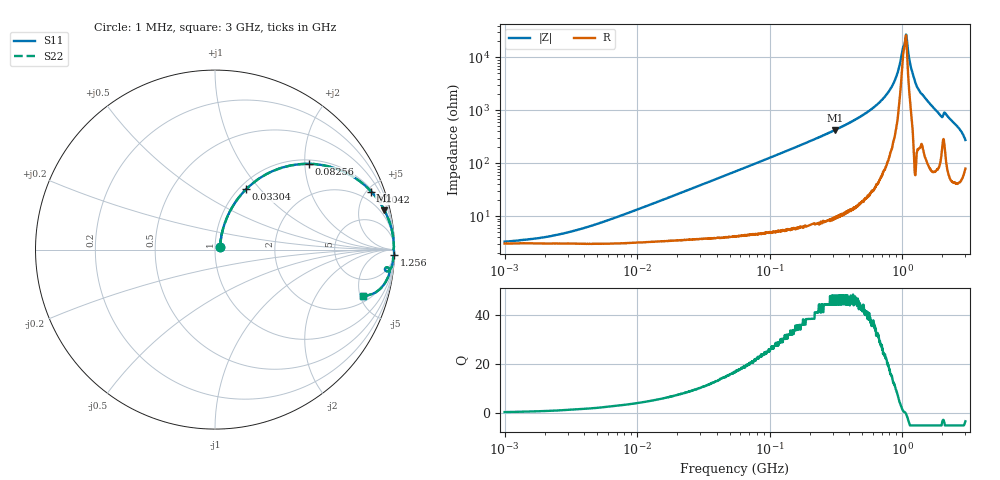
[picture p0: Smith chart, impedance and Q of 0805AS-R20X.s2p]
!s-Parameter Generated by FASTRON Sdn. Bhd.
!FASTRON P/N : 0805AS-R20X
!Keysight Technologies: E4991B_MY54100416_A.01.15
!Date: Mon Jun 15 12:52:56 2026
!Version  :Rev01  Mon Jun 15 12:52:56 2026
!Data & Calibration Information:
!Freq  S11  S21  S12  S22
!PortZ  Port1:50+j0  Port2:50+j0
!When reading reference impedance value at option line is always used.
! Remarks : This data is being provided solely for informational purposes.
# Hz S dB R 50
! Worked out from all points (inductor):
!   1601 points, 1 MHz to 3 GHz, reference 50 ohm
!   read as one part in series: L = 208 nH near 7.075 MHz
!   highest Q = 47.7 at 312.5 MHz (marker M1), where L = 218 nH
!   self-resonance near 1.059 GHz
!   S11 on the Smith chart (normalised r, x): 1 MHz: 1.06, +0.03; 33.04 MHz: 1.08, +0.85; 82.56 MHz: 1.09, +2.10; 204.2 MHz: 1.14, +5.32; 1.256 GHz: 2, -68; 3 GHz: 2.60, -5.30
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1000000  -29.80 22.4  -0.26 -0.7  -0.26 -0.7  -29.80 22.4
3804036  -24.90 55.9  -0.27 -2.8  -0.27 -2.8  -24.90 55.9
1.447069e7  -14.80 69.6  -0.43 -10.3  -0.43 -10.3  -14.80 69.6
3.304208e7  -8.41 62.7  -0.99 -22.2  -0.99 -22.2  -8.41 62.7
5.504702e7  -5.04 52.6  -1.98 -34.0  -1.98 -34.0  -5.04 52.6
8.255875e7  -2.98 42.3  -3.43 -45.1  -3.43 -45.1  -2.98 42.3
2.042267e8  -0.65 20.4  -9.15 -68.1  -9.15 -68.1  -0.65 20.4
2.083556e8  -0.62 20.0  -9.31 -68.5  -9.31 -68.5  -0.62 20.0
3.124888e8  -0.27 13.1  -12.90 -75.7  -12.90 -75.7  -0.27 13.1
5.611759e8  -0.07 5.8  -19.80 -82.7  -19.80 -82.7  -0.07 5.8
7.925923e8  -0.03 2.5  -27.20 -84.4  -27.20 -84.4  -0.03 2.5
9.117997e8  -0.02 1.2  -33.40 -82.1  -33.40 -82.1  -0.02 1.2
1.054198e9  -0.04 0.1  -46.60 -14.2  -46.60 -14.2  -0.04 0.1
1.091779e9  -0.03 -0.3  -45.50 56.0  -45.50 56.0  -0.03 -0.3
1.165162e9  -0.02 -0.9  -36.20 80.5  -36.20 80.5  -0.02 -0.9
1.255985e9  -0.01 -1.7  -30.60 87.3  -30.60 87.3  -0.01 -1.7
1.367504e9  -0.04 -2.6  -26.90 82.3  -26.90 82.3  -0.04 -2.6
1.738771e9  -0.09 -5.2  -20.90 81.2  -20.90 81.2  -0.09 -5.2
1.941122e9  -0.20 -6.9  -18.30 75.7  -18.30 75.7  -0.20 -6.9
2.145442e9  -0.19 -6.6  -18.70 76.1  -18.70 76.1  -0.19 -6.6
2.660507e9  -0.35 -11.7  -13.80 73.1  -13.80 73.1  -0.35 -11.7
3e9  -1.27 -17.4  -10.10 55.8  -10.10 55.8  -1.27 -17.4
